(* Logix 5000 AddOnInstructionDefinition export AOI_Weber_C30S_DN_Mapper; software revision 20.01 *)

TYPE UDT_PLC_To_C30S :   // Output from PLC
STRUCT
   Automatic : BOOL;
   Start : BOOL;
   AckFault : BOOL;
   DS1 : BOOL;
   DS2 : BOOL;
   ExtDigSig : BOOL;
   Res1 : BOOL;
   Res2 : BOOL;
   Prog : SINT;
END_STRUCT
END_TYPE

TYPE UDT_C30S_To_PLC :   // Input to PLC
STRUCT
   NoFault : BOOL;
   ReadyToStart : BOOL;
   OK : BOOL;
   NOK : BOOL;
   DepthReached : BOOL;
   Res1 : BOOL;
   Res2 : BOOL;
   Res3 : BOOL;
   ProgResult : SINT;
   StrategyResult : SINT;
   CodeResult : INT;
   TorqueResult : REAL;
   PreTorqueResult : REAL;
   AngleResult : REAL;
   DepthResult : REAL;
   DriveTime : REAL;
   CycleNumber : DINT;
END_STRUCT
END_TYPE

TYPE UDT_C30S_DN :   // In and Output Data for Weber C30S
STRUCT
   OUT : UDT_PLC_To_C30S;   // Output Data
   IN : UDT_C30S_To_PLC;   // Input Data
   Temp_In : SINT[29];
   Temp_Out : SINT[2];
END_STRUCT
END_TYPE

ADD_ON_INSTRUCTION AOI_Weber_C30S_DN_Mapper   (* revision 1.0, vendor Weber Schraubautomaten *)
// Maps DeviceNet IO Data to UDT_C30S
// Revision note:
// 18/02/2014 Create
VAR_IN_OUT
   Screwdriver_Data : UDT_C30S_DN; {required}
   Field_Inputs : SINT[29]; {required}   // Inputs from DeviceNet Scanner
   Field_Outputs : SINT[2]; {required}   // Outputs to DeviceNet Scanner
END_VAR
VAR
   TempReal : REAL; {access None}
   TempDint : DINT; {access None}
END_VAR

ROUTINE Logic   (* ladder *)
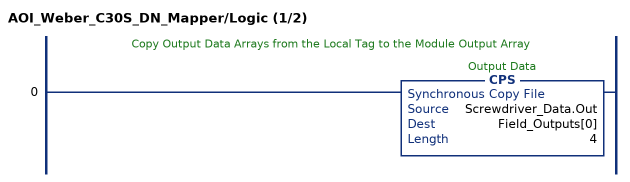
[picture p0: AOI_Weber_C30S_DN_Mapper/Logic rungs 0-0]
   // Copy Output Data Arrays from the Local Tag to the Module Output Array
   0: CPS(Screwdriver_Data.Out,Field_Outputs[0],4);
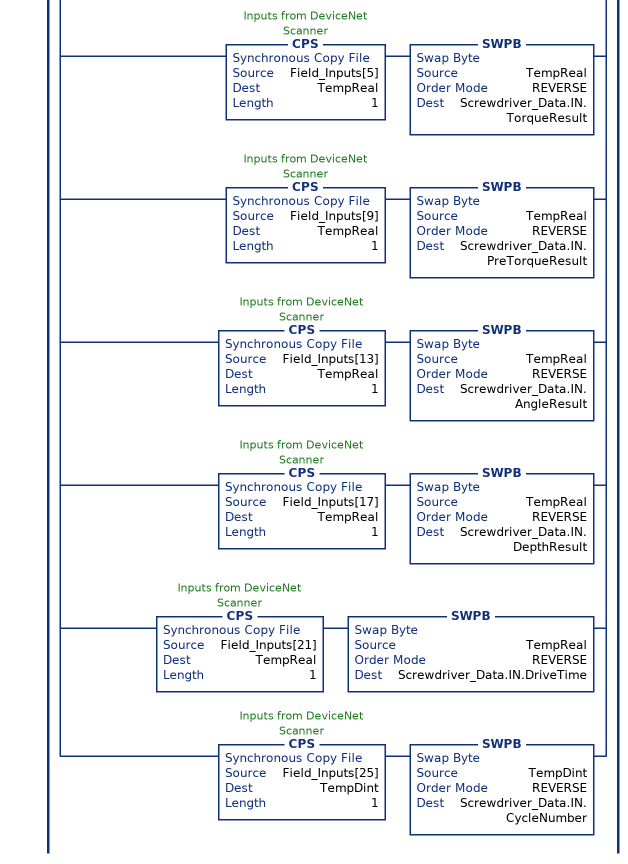
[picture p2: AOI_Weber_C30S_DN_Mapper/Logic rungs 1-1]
   // Map the Bit Signals of the SINT Array[0] to the Local Tags
   // Map the 2 Byte into the Tags Program and Strategy
   // Map the 2 Byte into the INT Tag CodeResult (Byte Swapping)
   // Map the last SINT into REAL and DINT Datatypes and perform the Byte-Swapping
   1: [XIC(Field_Inputs[0].0) OTE(Screwdriver_Data.IN.NoFault) ,XIC(Field_Inputs[0].1) OTE(Screwdriver_Data.IN.ReadyToStart) ,XIC(Field_Inputs[0].2) OTE(Screwdriver_Data.IN.OK) ,XIC(Field_Inputs[0].3) OTE(Screwdriver_Data.IN.NOK) ,XIC(Field_Inputs[0].4) OTE(Screwdriver_Data.IN.DepthReached) ,XIC(Field_Inputs[0].5) OTE(Screwdriver_Data.IN.Res1) ,XIC(Field_Inputs[0].6) OTE(Screwdriver_Data.IN.Res2) ,XIC(Field_Inputs[0].7) OTE(Screwdriver_Data.IN.Res3) ,CPS(Field_Inputs[1],Screwdriver_Data.IN.ProgResult,2) ,BTD(Field_Inputs[4],0,Screwdriver_Data.IN.CodeResult,0,8) BTD(Field_Inputs[3],0,Screwdriver_Data.IN.CodeResult,8,8) ,CPS(Field_Inputs[5],TempReal,1) SWPB(TempReal,REVERSE,Screwdriver_Data.IN.TorqueResult) ,CPS(Field_Inputs[9],TempReal,1) SWPB(TempReal,REVERSE,Screwdriver_Data.IN.PreTorqueResult) ,CPS(Field_Inputs[13],TempReal,1) SWPB(TempReal,REVERSE,Screwdriver_Data.IN.AngleResult) ,CPS(Field_Inputs[17],TempReal,1) SWPB(TempReal,REVERSE,Screwdriver_Data.IN.DepthResult) ,CPS(Field_Inputs[21],TempReal,1) SWPB(TempReal,REVERSE,Screwdriver_Data.IN.DriveTime) ,CPS(Field_Inputs[25],TempDint,1) SWPB(TempDint,REVERSE,Screwdriver_Data.IN.CycleNumber) ];
END_ROUTINE
END_ADD_ON_INSTRUCTION
